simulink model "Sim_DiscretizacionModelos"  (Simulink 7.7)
settings: Solver=ode45  StartTime=0.0  StopTime=8  RelTol=1e-13  AbsTol=1e-13
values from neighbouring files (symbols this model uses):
  a = T.f    [DiscretizacionModelos.m]
  b = T.b    [DiscretizacionModelos.m]
  Tc = tf(NUMc,DENc)    [DiscretizacionModelos.m]
  Ts = 0.3    [DiscretizacionModelos.m]

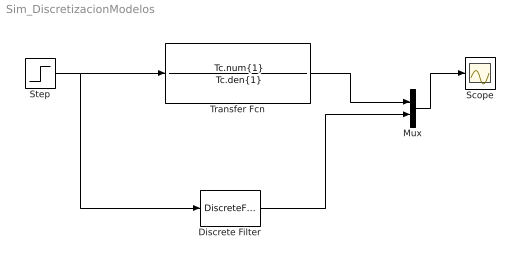
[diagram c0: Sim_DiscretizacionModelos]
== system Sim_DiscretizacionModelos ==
  Discrete Filter : DiscreteFilter  Numerator=b  Denominator=a  SampleTime=Ts
  Mux : Mux  Inputs=2
  Scope : Scope
  Step : Step  Time=0.1  SampleTime=0
  Transfer Fcn : TransferFcn  Numerator=Tc.num{1}  Denominator=Tc.den{1}
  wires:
  Step/1 -> Transfer Fcn/1, Discrete Filter/1
  Transfer Fcn/1 -> Mux/1
  Discrete Filter/1 -> Mux/2
  Mux/1 -> Scope/1
